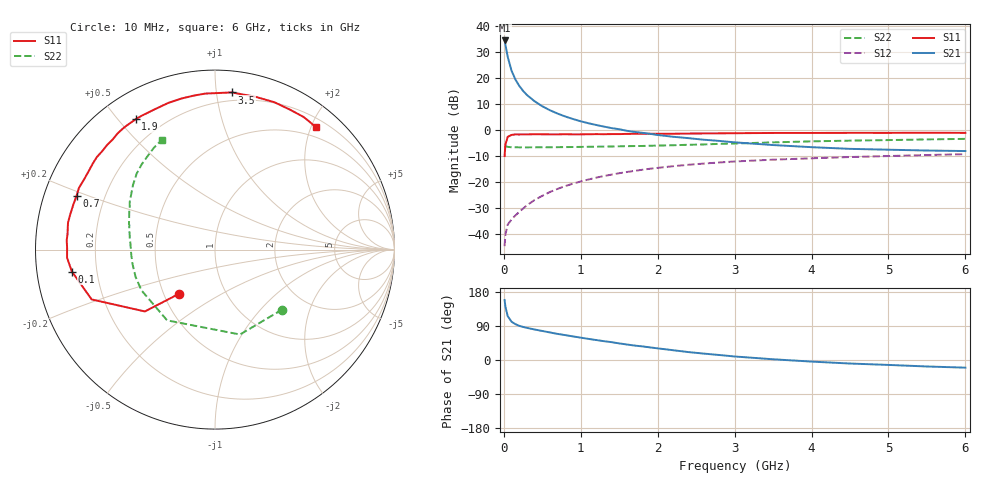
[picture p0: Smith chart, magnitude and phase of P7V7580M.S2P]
! SIEMENS Small Signal Semiconductors
! BFP196
! Si NPN RF Bipolar Junction Transistor in SOT143
! VCE = 0.75 V  IC = 80 mA
! Common Emitter S-Parameters:  May  1996
# GHz  S  MA  R  50
!  f  S11  S21  S12  S22
! GHz  MAG  ANG  MAG  ANG  MAG  ANG  MAG  ANG
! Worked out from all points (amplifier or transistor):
!   36 points, 10 MHz to 6 GHz, reference 50 ohm
!   highest |S21| = 34.4 dB at 10 MHz (marker M1)
!   |S21| within 3 dB of that: start of sweep to 29.29 MHz
!   unconditionally stable (mu >= 1): start of sweep to 11.97 MHz; 195.3 MHz to end of sweep
!   at 250 MHz: K = 1.08, MAG = 20.9 dB, |S12| = -30.1 dB
!   at 1.4 GHz: K = 1.20, MAG = 6.2 dB, |S12| = -17.1 dB
!   at 6 GHz: K = 1.08, MAG = -1.1 dB, |S12| = -9.2 dB
!   S11 on the Smith chart (normalised r, x): 10 MHz: 0.60, -0.33; 100 MHz: 0.11, -0.08; 700 MHz: 0.10, +0.19; 1.9 GHz: 0.11, +0.56; 3.5 GHz: 0.14, +1.10; 6 GHz: 0.33, +2.07
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0.01  0.3171 -129.1  52.63 158.4  0.0059 62.8  0.5018 -41.7
0.02  0.521 -138.6  44.12 141.3  0.0098 54.7  0.4932 -73.6
0.05  0.7411 -158.0  25.56 115.9  0.0153 42.0  0.476 -124.1
0.1  0.8069 -171.3  13.85 101.1  0.0192 43.9  0.4684 -150.9
0.15  0.8255 -176.9  9.387 94.6  0.0229 51.2  0.4679 -161.0
0.2  0.8239 179.4  7.088 90.2  0.0269 54.4  0.4656 -166.4
0.25  0.8279 176.3  5.663 87.2  0.0311 57.5  0.4666 -170.1
0.3  0.8263 174.0  4.723 84.8  0.036 60.7  0.4656 -172.3
0.4  0.8326 169.6  3.573 80.5  0.0455 62.6  0.4672 -175.7
0.5  0.83 166.2  2.868 76.6  0.0547 64.5  0.4679 -178.2
0.6  0.8281 162.3  2.4 72.7  0.0649 64.3  0.4682 179.9
0.7  0.8276 158.7  2.07 68.8  0.0745 63.9  0.47 178.3
0.9  0.8277 152.0  1.629 62.2  0.0937 62.1  0.4729 175.4
1.1  0.8323 145.1  1.354 55.7  0.1125 59.6  0.4781 172.9
1.6  0.8449 129.8  0.968 40.9  0.1567 51.6  0.4911 166.7
1.9  0.8501 121.3  0.848 33.3  0.1811 46.8  0.5008 163.2
2.2  0.8508 113.1  0.744 25.8  0.2026 41.6  0.5117 159.2
3  0.8709 93.6  0.582 9.3  0.2495 28.5  0.5526 148.3
3.5  0.8806 83.9  0.516 1.9  0.2704 21.2  0.5807 142.0
4.5  0.8853 68.0  0.436 -9.3  0.3038 8.7  0.6273 130.5
5.5  0.8887 56.2  0.405 -17.1  0.3322 -2.0  0.6618 120.9
6  0.8844 50.7  0.396 -20.2  0.3449 -7.8  0.6785 116.0
